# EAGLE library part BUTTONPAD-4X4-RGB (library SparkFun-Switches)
4x4 Button Pad w/ RGB LEDs Layout and schematic for 4x4 button pad with tri-color LEDs under each button. For use with the 4x Button Pad 2x2 - LED Compatible and 4x Button Pad 2x2 Top Bezel. Any RGB 5mm LED should be compatible. SparkFun Products SparkFun Simon Says - Through-Hole Soldering Kit (KIT-10547) Button Pad 2x2 - Breakout PCB (COM-09277)
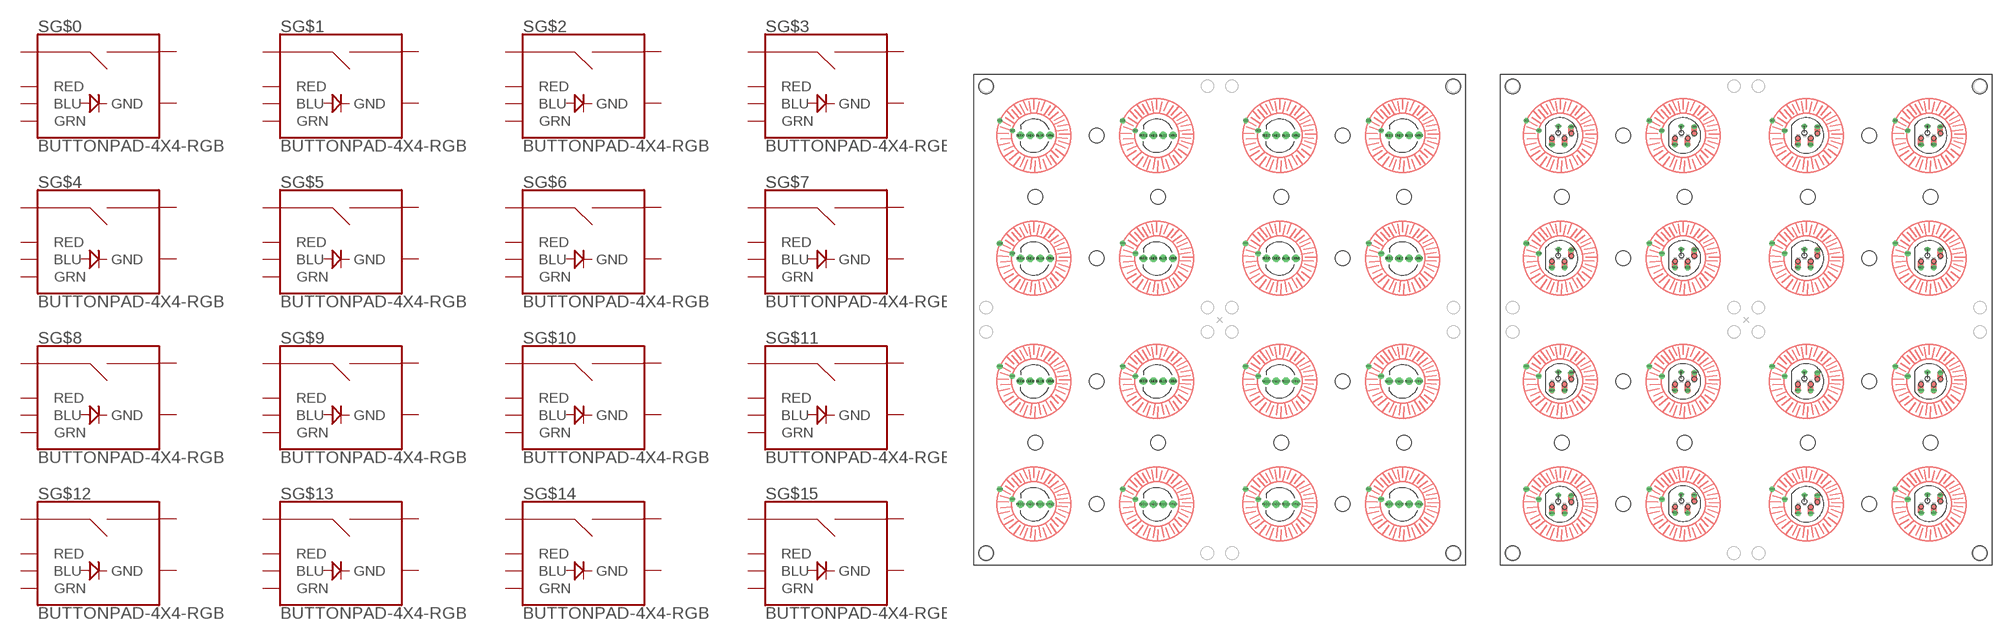
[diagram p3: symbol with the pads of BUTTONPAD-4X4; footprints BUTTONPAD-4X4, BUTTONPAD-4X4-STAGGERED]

Designator prefix S; gates G$0=BUTTONPAD-RGB G$1=BUTTONPAD-RGB G$2=BUTTONPAD-RGB G$3=BUTTONPAD-RGB G$4=BUTTONPAD-RGB G$5=BUTTONPAD-RGB G$6=BUTTONPAD-RGB G$7=BUTTONPAD-RGB G$8=BUTTONPAD-RGB G$9=BUTTONPAD-RGB G$10=BUTTONPAD-RGB G$11=BUTTONPAD-RGB G$12=BUTTONPAD-RGB G$13=BUTTONPAD-RGB G$14=BUTTONPAD-RGB G$15=BUTTONPAD-RGB

## BUTTONPAD-4X4-RGB (PROD_ID: COMP-08481; SF_SKU: COM-07836)  [BUTTONPAD-4X4]
BLU0  G$0:BLU
BLU1  G$1:BLU
BLU2  G$2:BLU
BLU3  G$3:BLU
BLU4  G$4:BLU
BLU5  G$5:BLU
BLU6  G$6:BLU
BLU7  G$7:BLU
BLU8  G$8:BLU
BLU9  G$9:BLU
BLU10  G$10:BLU
BLU11  G$11:BLU
BLU12  G$12:BLU
BLU13  G$13:BLU
BLU14  G$14:BLU
BLU15  G$15:BLU
GND0  G$0:GND
GND1  G$1:GND
GND2  G$2:GND
GND3  G$3:GND
GND4  G$4:GND
GND5  G$5:GND
GND6  G$6:GND
GND7  G$7:GND
GND8  G$8:GND
GND9  G$9:GND
GND10  G$10:GND
GND11  G$11:GND
GND12  G$12:GND
GND13  G$13:GND
GND14  G$14:GND
GND15  G$15:GND
GRN0  G$0:GRN
GRN1  G$1:GRN
GRN2  G$2:GRN
GRN3  G$3:GRN
GRN4  G$4:GRN
GRN5  G$6:GRN
GRN6  G$5:GRN
GRN7  G$7:GRN
GRN8  G$8:GRN
GRN9  G$9:GRN
GRN10  G$10:GRN
GRN11  G$11:GRN
GRN12  G$12:GRN
GRN13  G$13:GRN
GRN14  G$14:GRN
GRN15  G$15:GRN
RED0  G$0:RED
RED1  G$1:RED
RED2  G$2:RED
RED3  G$3:RED
RED4  G$4:RED
RED5  G$5:RED
RED6  G$6:RED
RED7  G$7:RED
RED8  G$8:RED
RED9  G$9:RED
RED10  G$10:RED
RED11  G$11:RED
RED12  G$12:RED
RED13  G$13:RED
RED14  G$14:RED
RED15  G$15:RED
SIG0  G$0:SIG1
SIG1  G$0:SIG2
SIG2  G$1:SIG1
SIG3  G$1:SIG2
SIG4  G$2:SIG1
SIG5  G$2:SIG2
SIG6  G$3:SIG1
SIG7  G$3:SIG2
SIG8  G$4:SIG1
SIG9  G$4:SIG2
SIG10  G$5:SIG1
SIG11  G$5:SIG2
SIG12  G$6:SIG1
SIG13  G$6:SIG2
SIG14  G$7:SIG1
SIG15  G$7:SIG2
SIG16  G$8:SIG1
SIG17  G$8:SIG2
SIG18  G$9:SIG1
SIG19  G$9:SIG2
SIG20  G$10:SIG1
SIG21  G$10:SIG2
SIG22  G$11:SIG1
SIG23  G$11:SIG2
SIG24  G$12:SIG1
SIG25  G$12:SIG2
SIG26  G$13:SIG1
SIG27  G$13:SIG2
SIG28  G$14:SIG1
SIG29  G$14:SIG2
SIG30  G$15:SIG1
SIG31  G$15:SIG2

## BUTTONPAD-4X4-RGB-STAGGERED (PROD_ID: COMP-08481; SF_SKU: COM-07836)  [BUTTONPAD-4X4-STAGGERED]
Pads as for BUTTONPAD-4X4

## Footprint BUTTONPAD-4X4 (pad centres in mm)
4x4 Button Pad w/ RGB LEDs Layout and schematic for 4x4 button pad with tri-color LEDs under each button. For use with the 4x Button Pad 2x2 - LED Compatible and 4x Button Pad 2x2 Top Bezel. Any RGB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
drill 1: BLU0 13.5,87.5; BLU1 38.5,87.5; BLU2 63.5,87.5; BLU3 88.5,87.5; BLU4 13.5,62.5; BLU5 38.5,62.5; BLU6 63.5,62.5; BLU7 88.5,62.5; BLU8 13.5,37.5; BLU9 38.5,37.5; BLU10 63.5,37.5; BLU11 88.5,37.5; BLU12 13.5,12.5; BLU13 38.5,12.5; BLU14 63.5,12.5; BLU15 88.5,12.5; GND0 11.5,87.5; GND1 36.5,87.5; GND2 61.5,87.5; GND3 86.5,87.5; GND4 11.5,62.5; GND5 36.5,62.5; GND6 61.5,62.5; GND7 86.5,62.5; GND8 11.5,37.5; GND9 36.5,37.5; GND10 61.5,37.5; GND11 86.5,37.5; GND12 11.5,12.5; GND13 36.5,12.5; GND14 61.5,12.5; GND15 86.5,12.5; GRN0 15.5,87.5; GRN1 40.5,87.5; GRN2 65.5,87.5; GRN3 90.5,87.5; GRN4 15.5,62.5; GRN5 40.5,62.5; GRN6 65.5,62.5; GRN7 90.5,62.5; GRN8 15.5,37.5; GRN9 40.5,37.5; GRN10 65.5,37.5; GRN11 90.5,37.5; GRN12 15.5,12.5; GRN13 40.5,12.5; GRN14 65.5,12.5; GRN15 90.5,12.5; RED0 9.5,87.5; RED1 34.5,87.5; RED2 59.5,87.5; RED3 84.5,87.5; RED4 9.5,62.5; RED5 34.5,62.5; RED6 59.5,62.5; RED7 84.5,62.5; RED8 9.5,37.5; RED9 34.5,37.5; RED10 59.5,37.5; RED11 84.5,37.5; RED12 9.5,12.5; RED13 34.5,12.5; RED14 59.5,12.5; RED15 84.5,12.5
drill 0.508: SIG0 5.288,90.513; SIG1 7.828,88.481; SIG2 30.288,90.513; SIG3 32.828,88.481; SIG4 55.288,90.513; SIG5 57.828,88.481; SIG6 80.288,90.513; SIG7 82.828,88.481
drill 0.6: SIG8 5.288,65.513; SIG9 7.828,63.481; SIG10 30.288,65.513; SIG11 32.828,63.481; SIG12 55.288,65.513; SIG13 57.828,63.481; SIG14 80.288,65.513; SIG15 82.828,63.481; SIG16 5.288,40.513; SIG17 7.828,38.481; SIG18 30.288,40.513; SIG19 32.828,38.481; SIG20 55.288,40.513; SIG21 57.828,38.481; SIG22 80.288,40.513; SIG23 82.828,38.481; SIG24 5.288,15.513; SIG25 7.828,13.481; SIG26 30.288,15.513; SIG27 32.828,13.481; SIG28 55.288,15.513; SIG29 57.828,13.481; SIG30 80.288,15.513; SIG31 82.828,13.481
hole 3 at 12.5,25
hole 3 at 25,37.5
hole 3 at 37.5,25
hole 3 at 25,12.5
hole 3 at 62.5,25
hole 3 at 75,37.5
hole 3 at 87.5,25
hole 3 at 75,12.5
hole 3 at 12.5,75
hole 3 at 25,87.5
hole 3 at 37.5,75
hole 3 at 25,62.5
hole 3 at 62.5,75
hole 3 at 75,87.5
hole 3 at 87.5,75
hole 3 at 75,62.5
hole 3 at 2.484,97.516
hole 3 at 97.516,97.516
hole 3 at 97.516,2.484
hole 3 at 2.484,2.484

## Footprint BUTTONPAD-4X4-STAGGERED (pad centres in mm)
4x4 Button Pad w/ RGB LEDs - Staggered LED Footprint Layout and schematic for 4x4 button pad with tri-color LEDs under each button. For use with the 4x Button Pad 2x2 - LED Compatible and 4x Button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
drill 0.508: BLU0 13.081,85.623; BLU1 38.1,85.623; BLU2 63.119,85.623; BLU3 88.138,85.623; BLU4 13.081,60.604; BLU5 38.1,60.604; BLU6 63.119,60.604; BLU7 88.138,60.604; BLU8 13.081,35.585; BLU9 38.1,35.585; BLU10 63.119,35.585; BLU11 88.138,35.585; BLU12 13.081,10.566; BLU13 38.1,10.693; BLU14 63.119,10.566; BLU15 88.138,10.693; GND0 11.786,89.357; GND1 36.805,89.357; GND2 61.824,89.357; GND3 86.843,89.357; GND4 11.786,64.338; GND5 36.805,64.338; GND6 61.824,64.338; GND7 86.843,64.338; GND8 11.786,39.319; GND9 36.805,39.319; GND10 61.824,39.319; GND11 86.843,39.319; GND12 11.786,14.3; GND13 36.805,14.427; GND14 61.824,14.3; GND15 86.843,14.427; GRN0 14.427,89.256; GRN1 39.446,89.256; GRN2 64.465,89.256; GRN3 89.484,89.256; GRN4 14.427,64.237; GRN5 39.446,64.237; GRN6 64.465,64.237; GRN7 89.484,64.237; GRN8 14.427,39.218; GRN9 39.446,39.218; GRN10 64.465,39.218; GRN11 89.484,39.218; GRN12 14.427,14.199; GRN13 39.446,14.326; GRN14 64.465,14.199; GRN15 89.484,14.326; RED0 10.49,85.623; RED1 35.509,85.623; RED2 60.528,85.623; RED3 85.547,85.623; RED4 10.49,60.604; RED5 35.509,60.604; RED6 60.528,60.604; RED7 85.547,60.604; RED8 10.49,35.585; RED9 35.509,35.585; RED10 60.528,35.585; RED11 85.547,35.585; RED12 10.49,10.566; RED13 35.509,10.693; RED14 60.528,10.566; RED15 85.547,10.693; SIG0 5.288,90.513; SIG1 7.828,88.481; SIG2 30.288,90.513; SIG3 32.828,88.481; SIG4 55.288,90.513; SIG5 57.828,88.481; SIG6 80.288,90.513; SIG7 82.828,88.481
drill 0.6: SIG8 5.288,65.513; SIG9 7.828,63.481; SIG10 30.288,65.513; SIG11 32.828,63.481; SIG12 55.288,65.513; SIG13 57.828,63.481; SIG14 80.288,65.513; SIG15 82.828,63.481; SIG16 5.288,40.513; SIG17 7.828,38.481; SIG18 30.288,40.513; SIG19 32.828,38.481; SIG20 55.288,40.513; SIG21 57.828,38.481; SIG22 80.288,40.513; SIG23 82.828,38.481; SIG24 5.288,15.513; SIG25 7.828,13.481; SIG26 30.288,15.513; SIG27 32.828,13.481; SIG28 55.288,15.513; SIG29 57.828,13.481; SIG30 80.288,15.513; SIG31 82.828,13.481
hole 3 at 12.5,25
hole 3 at 25,37.5
hole 3 at 37.5,25
hole 3 at 25,12.5
hole 3 at 62.5,25
hole 3 at 75,37.5
hole 3 at 87.5,25
hole 3 at 75,12.5
hole 3 at 12.5,75
hole 3 at 25,87.5
hole 3 at 37.5,75
hole 3 at 25,62.5
hole 3 at 62.5,75
hole 3 at 75,87.5
hole 3 at 87.5,75
hole 3 at 75,62.5
hole 3 at 2.484,97.516
hole 3 at 97.516,97.516
hole 3 at 97.516,2.484
hole 3 at 2.484,2.484
hole 0.914 at 10.49,86.919
hole 0.914 at 11.786,88.062
hole 0.914 at 13.081,86.919
hole 0.914 at 14.427,87.96
hole 0.914 at 35.509,86.919
hole 0.914 at 36.805,88.062
hole 0.914 at 38.1,86.919
hole 0.914 at 39.446,87.96
hole 0.914 at 60.528,86.919
hole 0.914 at 61.824,88.062
hole 0.914 at 63.119,86.919
hole 0.914 at 64.465,87.96
hole 0.914 at 85.547,86.919
hole 0.914 at 86.843,88.062
hole 0.914 at 88.138,86.919
hole 0.914 at 89.484,87.96
hole 0.914 at 10.49,61.9
hole 0.914 at 11.786,63.043
hole 0.914 at 13.081,61.9
hole 0.914 at 14.427,62.941
hole 0.914 at 35.509,61.9
hole 0.914 at 36.805,63.043
hole 0.914 at 38.1,61.9
hole 0.914 at 39.446,62.941
hole 0.914 at 60.528,61.9
hole 0.914 at 61.824,63.043
hole 0.914 at 63.119,61.9
hole 0.914 at 64.465,62.941
hole 0.914 at 85.547,61.9
hole 0.914 at 86.843,63.043
hole 0.914 at 88.138,61.9
hole 0.914 at 89.484,62.941
hole 0.914 at 10.49,36.881
hole 0.914 at 11.786,38.024
hole 0.914 at 13.081,36.881
hole 0.914 at 14.427,37.922
hole 0.914 at 35.509,36.881
hole 0.914 at 36.805,38.024
hole 0.914 at 38.1,36.881
hole 0.914 at 39.446,37.922
hole 0.914 at 60.528,36.881
hole 0.914 at 61.824,38.024
hole 0.914 at 63.119,36.881
hole 0.914 at 64.465,37.922
hole 0.914 at 85.547,36.881
hole 0.914 at 86.843,38.024
hole 0.914 at 88.138,36.881
hole 0.914 at 89.484,37.922
hole 0.914 at 10.49,11.862
hole 0.914 at 11.786,13.005
hole 0.914 at 13.081,11.862
hole 0.914 at 14.427,12.903
hole 0.914 at 35.509,11.989
hole 0.914 at 36.805,13.132
hole 0.914 at 38.1,11.989
hole 0.914 at 39.446,13.03
hole 0.914 at 60.528,11.862
hole 0.914 at 61.824,13.005
hole 0.914 at 63.119,11.862
hole 0.914 at 64.465,12.903
hole 0.914 at 85.547,11.989
hole 0.914 at 86.843,13.132
hole 0.914 at 88.138,11.989
hole 0.914 at 89.484,13.03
